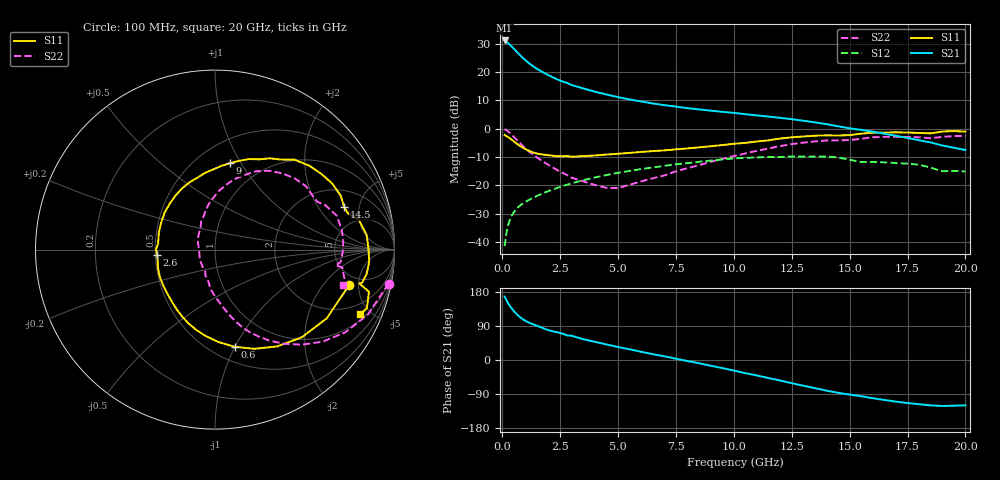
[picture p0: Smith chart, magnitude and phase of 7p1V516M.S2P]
! Infineon Technologies  Discrete & RF Semiconductors
! bfp620
! VCE =  1.5 V,  IC =  16 mA
! Common Emitter S-Parameters:  Sep 2002
# GHz  S  MA  R  50
!  f  S11  S21  S12  S22
! GHz  MAG  ANG  MAG  ANG  MAG  ANG  MAG  ANG
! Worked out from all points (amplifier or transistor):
!   59 points, 100 MHz to 20 GHz, reference 50 ohm
!   highest |S21| = 31.2 dB at 100 MHz (marker M1)
!   |S21| within 3 dB of that: start of sweep to 507.4 MHz
!   unconditionally stable (mu >= 1): 3.682 GHz to 10.01 GHz; 17.13 GHz to end of sweep
!   at 1 GHz: K = 0.62, MSG = 25.0 dB, |S12| = -25.9 dB
!   at 5.5 GHz: K = 1.04, MAG = 11.4 dB, |S12| = -14.9 dB
!   at 20 GHz: K = 1.34, MAG = 0.3 dB, |S12| = -15.1 dB
!   S11 on the Smith chart (normalised r, x): 100 MHz: 3.89, -3.83; 600 MHz: 0.64, -1.00; 2.6 GHz: 0.51, -0.03; 9 GHz: 0.71, +0.90; 14.5 GHz: 3.15, +3.52; 20 GHz: 1.29, -4.34
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0.1  0.7724 -14.9  36.12 167.5  0.0084 82.3  0.9856 -11.1
0.2  0.7309 -31.6  33.62 155.2  0.0163 75.2  0.9264 -22.9
0.3  0.6875 -45.3  31.03 145.1  0.023 69.9  0.8603 -32.4
0.4  0.6409 -57.3  28.36 136.5  0.0286 65.7  0.7894 -40.5
0.5  0.5949 -68.3  25.76 129.0  0.0335 62.3  0.7184 -47.5
0.6  0.5529 -78.4  23.33 122.3  0.0377 59.5  0.6512 -53.7
0.7  0.5163 -87.6  21.15 116.4  0.0415 57.4  0.5902 -59.2
0.9  0.4583 -103.5  17.57 107.0  0.048 54.6  0.4891 -68.0
1  0.4354 -110.2  16.14 103.3  0.0509 53.7  0.4482 -71.4
1.2  0.3985 -121.6  13.84 97.5  0.0564 52.4  0.3818 -76.8
1.5  0.3632 -136.1  11.39 90.3  0.0648 51.0  0.3092 -83.5
1.9  0.3432 -152.9  9.221 80.7  0.0763 49.2  0.2417 -92.8
2.6  0.3239 -175.0  6.807 69.5  0.0964 45.4  0.1657 -105.4
3.5  0.3272 163.1  5.128 54.8  0.1231 38.9  0.1173 -126.5
5  0.3597 134.3  3.606 34.3  0.1659 26.4  0.0892 176.0
7  0.4127 103.6  2.599 9.7  0.2204 8.3  0.1491 122.4
9  0.4894 80.1  2.08 -15.0  0.2728 -12.1  0.2596 97.1
10.5  0.5609 63.7  1.801 -34.8  0.3051 -30.1  0.3645 80.5
13.5  0.75 29.3  1.29 -74.2  0.3223 -65.2  0.5949 42.0
14.5  0.7578 18.3  1.101 -86.6  0.3098 -80.2  0.621 29.0
17  0.8618 -4.6  0.75 -109.8  0.2475 -96.5  0.716 3.6
20  0.8865 -24.0  0.42 -119.6  0.1752 -107.3  0.742 -15.5
